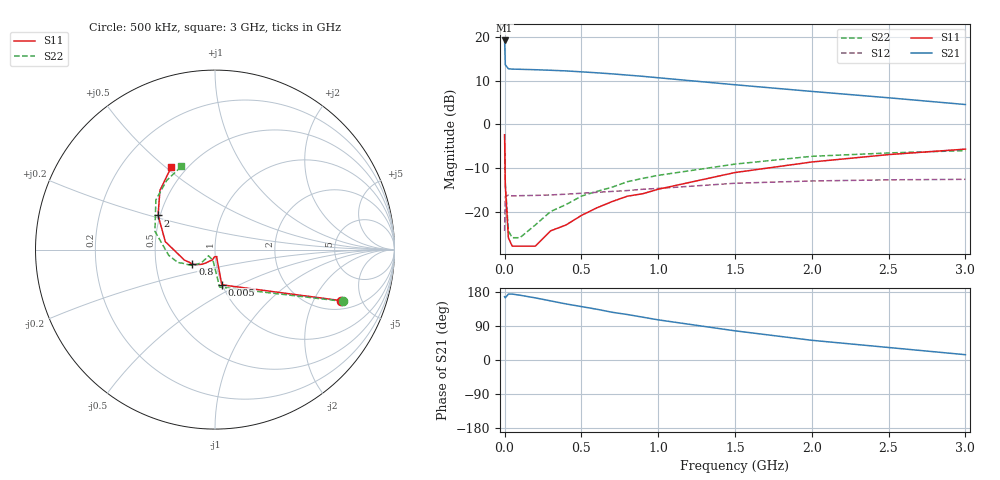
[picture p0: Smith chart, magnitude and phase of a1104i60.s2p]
!  MSA-1104 S AND NOISE PARAMETERS
!  Id=60mA  LAST UPDATED 07-27-92
# ghz s ma r 50
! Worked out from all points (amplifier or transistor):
!   18 points, 500 kHz to 3 GHz, reference 50 ohm
!   highest |S21| = 19.3 dB at 500 kHz (marker M1)
!   |S21| within 3 dB of that: start of sweep to 2.916 MHz
!   unconditionally stable (mu >= 1): 9.669 MHz to 1.476 GHz; 2.015 GHz to end of sweep
!   at 50 MHz: K = 1.09, MAG = 12.7 dB, |S12| = -16.4 dB
!   at 600 MHz: K = 1.06, MAG = 12.3 dB, |S12| = -15.6 dB
!   at 3 GHz: K = 1.05, MAG = 7.2 dB, |S12| = -12.6 dB
!   lowest NFmin = 3.40 dB at 100 MHz
!   S11 on the Smith chart (normalised r, x): 500 kHz: 2.51, -3.38; 5 MHz: 1.00, -0.41; 800 MHz: 0.77, -0.13; 2 GHz: 0.49, +0.22; 3 GHz: 0.41, +0.52
0.0005  0.76 -22.0  9.19 167.0  0.06 54.0  0.77 -22.0
0.005  0.2 -79.0  4.83 164.0  0.149 12.0  0.21 -83.0
0.025  0.05 -78.0  4.35 174.0  0.154 2.0  0.06 -101.0
0.05  0.04 -75.0  4.31 174.0  0.151 2.0  0.05 -136.0
0.1  0.04 -81.0  4.29 171.0  0.152 2.0  0.05 -137.0
0.2  0.04 -93.0  4.24 164.0  0.153 3.0  0.07 -135.0
0.3  0.06 -105.0  4.18 156.0  0.155 4.0  0.1 -136.0
0.4  0.07 -115.0  4.11 148.0  0.158 5.0  0.12 -139.0
0.5  0.09 -124.0  4.01 141.0  0.162 6.0  0.15 -144.0
0.6  0.11 -132.0  3.91 134.0  0.166 7.0  0.17 -150.0
0.7  0.13 -140.0  3.8 126.0  0.17 7.0  0.19 -156.0
0.8  0.15 -147.0  3.68 120.0  0.174 7.0  0.22 -161.0
0.9  0.16 -154.0  3.56 113.0  0.18 7.0  0.24 -168.0
1  0.18 -161.0  3.43 106.0  0.184 6.0  0.26 -173.0
1.5  0.28 171.0  2.85 77.0  0.211 2.0  0.35 163.0
2  0.37 149.0  2.39 52.0  0.224 -5.0  0.43 140.0
2.5  0.45 133.0  2.02 33.0  0.231 -10.0  0.47 125.0
3  0.52 118.0  1.69 14.0  0.234 -16.0  0.5 112.0
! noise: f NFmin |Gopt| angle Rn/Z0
0.1  3.4  0.02  11  0.43
0.5  3.6  0.02  102  0.42
1  4.1  0.06  168  0.41
2  5.4  0.17  -138  0.44
